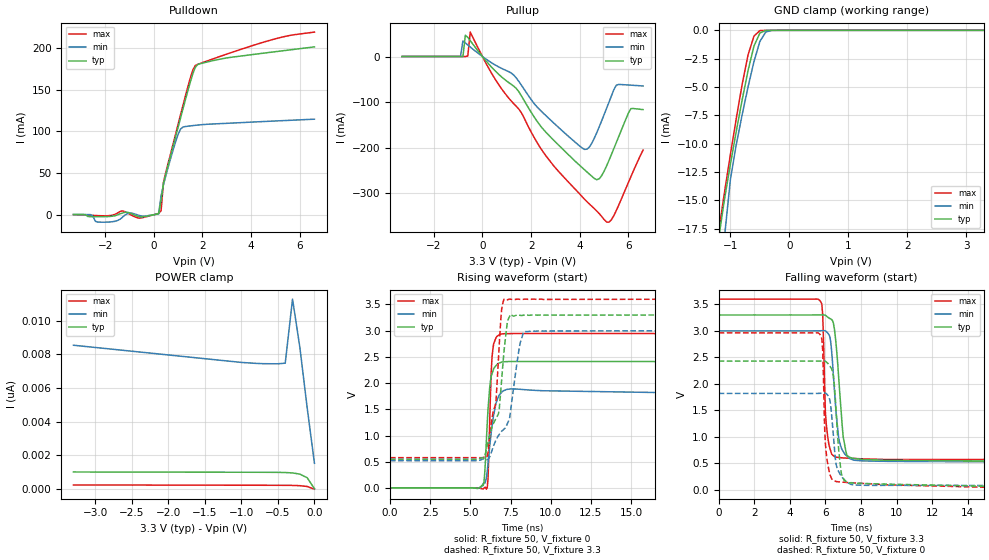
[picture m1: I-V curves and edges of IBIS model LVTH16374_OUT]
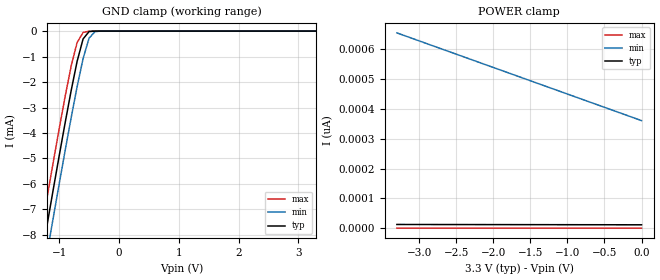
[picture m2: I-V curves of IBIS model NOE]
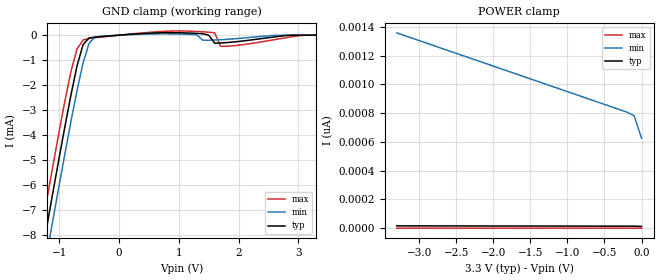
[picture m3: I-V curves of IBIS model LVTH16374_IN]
|   TEXAS INSTRUMENTS INCORPORATED
|   Standard Linear and Logic
|   IBIS Model of SN74LVTH16374
|   3.3V ABT 16-BIT  EDGE-TRIGGERED D-TYPE FLIP-FLOPS
|   WITH 3-STATE OUTPUTS
|   SSOP 48 PIN PACKAGE (DL)
|   TSSOP 48 PIN PACKAGE (DGG)
[IBIS Ver]   2.1
[Comment char]   |_char
[File Name]   sn74lvth16374.ibs
[File Rev]   1.0
[Date]   06-12-2000
[Source]   Data created from HSPICE simulations at TI ,SLL.
[Notes]   The following is an IBIS list for LVTH16374
   - All test data contained in this file are derived from hspice
   (tm) simulations.
   - This file may be incomplete or may not be fully compliant
   with the IBIS specification. It will be replaced with a
   version that is IBIS Revision 3.2 compliant and is complete
   and accurate. Please email all questions and comments to
   sllibis@ti.com.
|   -For Questions or Comments please mailto:sllibis@ti.com
|  [Disclaimer]
|*   Property of Texas Instruments Incorporated.  Unauthorized   *
|*   reproduction and/or distribution is strictly prohibited.   *
|*   This product is protected under copyright law.   *
|*   Created 1995, (C) Copyright 1995, Texas Instruments Inc.,   *
|*   All Rights Reserved   *
|*   UNLESS THERE IS A SIGNED, WRITTEN AGREEMENT TO THE   *
|*   CONTRARY, TEXAS INSTRUMENTS ("TI") IS PROVIDING THE SPICE   *
|*   MODELS "AS IS" AND WITHOUT ANY WARRANTY, EXPRESSED OR   *
|*   IMPLIED.  TI assumes no liability for:   *
|*   1) the accuracy of the IBIS models provided to your   *
|*   company;   *
|*   2) the proper functioning of these IBIS models in your   *
|*   design or for any resulting applications; or   *
|*   3) infringement of patents, copyrights or intellectual   *
|*   property rights resulting from your use of these   *
|*   IBIS models.   *
|*   TI provides IBIS Models as a service to our customers.   *
|*   You and your company shall not distribute, sell or give   *
|*   these models to anyone else without prior written   *
|*   permission from TI.   *
|*   TI reserves the right to make changes to our products or   *
|*   to discontinue any semiconductor product or service   *
|*   without notice, and advises our customers to obtain the   *
|*   latest version of relevant information to verify, before   *
|*   placing orders, that the information being relied on is   *
|*   current.   *
|*   Please be aware that your receipt and use of the IBIS   *
|*   information provided shall serve as acceptance of these   *
|*   terms and conditions.  If you do not accept these terms,   *
|*   you should return or destroy the IBIS models and any   *
|*   other accompanying information immediately.   *
[Component]   LVTH16374_DL
[manufacturer]   Texas   Instruments,   Inc.
[Package]
|   typ   min   max
R_pkg   0.048   0.038   0.053
L_pkg   6.046nH   5.084nH   7.968nH
C_pkg   0.813pF   0.569pF   1.157pF
[Pin]   signal_name   model_name   R_pin   L_pin   C_pin
1   1NOE   NOE   0.046   7.968nH   1.017pF
2   1Q1   LVTH16374_OUT   0.044   7.299nH   1.157pF
3   1Q2   LVTH16374_OUT   0.043   6.765nH   1.058pF
4   GND   GND   0.041   6.269nH   0.933pF
5   1Q3   LVTH16374_OUT   0.038   5.856nH   0.829pF
6   1Q4   LVTH16374_OUT   0.046   5.802nH   0.79pF
7   VCC   POWER   0.05   5.656nH   0.738pF
8   1Q5   LVTH16374_OUT   0.053   5.5nH   0.643pF
9   1Q6   LVTH16374_OUT   0.052   5.304nH   0.606pF
10   GND   GND   0.053   5.189nH   0.583pF
11   1Q7   LVTH16374_OUT   0.051   5.084nH   0.569pF
12   1Q8   LVTH16374_OUT   0.053   5.862nH   0.833pF
13   2Q1   LVTH16374_OUT   0.053   5.862nH   0.833pF
14   2Q2   LVTH16374_OUT   0.051   5.084nH   0.569pF
15   GND   GND   0.053   5.189nH   0.583pF
16   2Q3   LVTH16374_OUT   0.052   5.304nH   0.606pF
17   2Q4   LVTH16374_OUT   0.053   5.5nH   0.643pF
18   VCC   POWER   0.05   5.656nH   0.738pF
19   2Q5   LVTH16374_OUT   0.046   5.802nH   0.79pF
20   2Q6   LVTH16374_OUT   0.038   5.856nH   0.829pF
21   GND   GND   0.041   6.269nH   0.933pF
22   2Q7   LVTH16374_OUT   0.043   6.765nH   1.058pF
23   2Q8   LVTH16374_OUT   0.044   7.299nH   1.157pF
24   2NOE   NOE   0.046   7.968nH   1.017pF
25   2CLK   CLK   0.046   7.968nH   1.017pF
26   2D8   LVTH16374_IN   0.044   7.299nH   1.157pF
27   2D7   LVTH16374_IN   0.043   6.765nH   1.058pF
28   GND   GND   0.041   6.269nH   0.933pF
29   2D6   LVTH16374_IN   0.038   5.856nH   0.829pF
30   2D5   LVTH16374_IN   0.046   5.802nH   0.79pF
31   VCC   POWER   0.05   5.656nH   0.738pF
32   2D4   LVTH16374_IN   0.053   5.5nH   0.643pF
33   2D3   LVTH16374_IN   0.052   5.304nH   0.606pF
34   GND   LVTH16374_IN   0.053   5.189nH   0.583pF
35   2D2   LVTH16374_IN   0.051   5.084nH   0.569pF
36   2D1   LVTH16374_IN   0.053   5.862nH   0.833pF
37   1D8   LVTH16374_IN   0.053   5.862nH   0.833pF
38   1D7   LVTH16374_IN   0.051   5.084nH   0.569pF
39   GND   GND   0.053   5.189nH   0.583pF
40   1D6   LVTH16374_IN   0.052   5.304nH   0.606pF
41   1D5   LVTH16374_IN   0.053   5.5nH   0.643pF
42   VCC   POWER   0.05   5.656nH   0.738pF
43   1D4   LVTH16374_IN   0.046   5.802nH   0.79pF
44   1D3   LVTH16374_IN   0.038   5.856nH   0.829pF
45   GND   GND   0.041   6.269nH   0.933pF
46   1D2   LVTH16374_IN   0.043   6.765nH   1.058pF
47   1D1   LVTH16374_IN   0.044   7.299nH   1.157pF
48   1CLK   CLK   0.046   7.967nH   1.017pF
[Component]   LVTH16374_DGG
[manufacturer]   Texas   Instruments,   Inc.
[Package]
|   typ   min   max
R_pkg   0.056   0.039   0.068
L_pkg   3.39nH   3.078nH   3.995nH
C_pkg   0.52pF   0.414pF   0.668pF
[Pin]   signal_name   model_name   R_pin   L_pin   C_pin
1   1NOE   NOE   0.039   3.987nH   0.654pF
2   1Q1   LVTH16374_OUT   0.047   3.725nH   0.659pF
3   1Q2   LVTH16374_OUT   0.059   3.692nH   0.604pF
4   GND   GND   0.068   3.675nH   0.606pF
5   1Q3   LVTH16374_OUT   0.055   3.473nH   0.547pF
6   1Q4   LVTH16374_OUT   0.056   3.402nH   0.497pF
7   VCC   POWER   0.057   3.3nH   0.492pF
8   1Q5   LVTH16374_OUT   0.056   3.189nH   0.455pF
9   1Q6   LVTH16374_OUT   0.058   3.154nH   0.449pF
10   GND   GND   0.058   3.094nH   0.436pF
11   1Q7   LVTH16374_OUT   0.058   3.078nH   0.424pF
12   1Q8   LVTH16374_OUT   0.06   3.081nH   0.414pF
13   2Q1   LVTH16374_OUT   0.061   3.097nH   0.416pF
14   2Q2   LVTH16374_OUT   0.06   3.126nH   0.427pF
15   GND   GND   0.061   3.158nH   0.44pF
16   2Q3   LVTH16374_OUT   0.058   3.173nH   0.45pF
17   2Q4   LVTH16374_OUT   0.056   3.189nH   0.455pF
18   VCC   POWER   0.056   3.265nH   0.49pF
19   2Q5   LVTH16374_OUT   0.054   3.322nH   0.492pF
20   2Q6   LVTH16374_OUT   0.052   3.388nH   0.544pF
21   GND   GND   0.064   3.591nH   0.605pF
22   2Q7   LVTH16374_OUT   0.059   3.677nH   0.612pF
23   2Q8   LVTH16374_OUT   0.046   3.678nH   0.668pF
24   2NOE   NOE   0.041   3.979nH   0.659pF
25   2CLK   CLK   0.04   3.995nH   0.658pF
26   2D8   LVTH16374_IN   0.046   3.69nH   0.662pF
27   2D7   LVTH16374_IN   0.057   3.649nH   0.602pF
28   GND   GND   0.066   3.615nH   0.602pF
29   2D6   LVTH16374_IN   0.055   3.447nH   0.547pF
30   2D5   LVTH16374_IN   0.054   3.326nH   0.492pF
31   VCC   POWER   0.055   3.239nH   0.488pF
32   2D4   LVTH16374_IN   0.056   3.183nH   0.454pF
33   2D3   LVTH16374_IN   0.057   3.144nH   0.447pF
34   GND   LVTH16374_IN   0.058   3.099nH   0.436pF
35   2D2   LVTH16374_IN   0.059   3.086nH   0.425pF
36   2D1   LVTH16374_IN   0.06   3.081nH   0.414pF
37   1D8   LVTH16374_IN   0.061   3.097nH   0.415pF
38   1D7   LVTH16374_IN   0.06   3.119nH   0.427pF
39   GND   GND   0.06   3.144nH   0.439pF
40   1D6   LVTH16374_IN   0.056   3.13nH   0.446pF
41   1D5   LVTH16374_IN   0.057   3.208nH   0.456pF
42   VCC   POWER   0.056   3.247nH   0.487pF
43   1D4   LVTH16374_IN   0.054   3.328nH   0.491pF
44   1D3   LVTH16374_IN   0.053   3.413nH   0.546pF
45   GND   GND   0.066   3.609nH   0.606pF
46   1D2   LVTH16374_IN   0.058   3.689nH   0.607pF
47   1D1   LVTH16374_IN   0.047   3.727nH   0.662pF
48   1CLK   CLK   0.04   3.978nH   0.655pF
| Models and submodels in the file (4): LVTH16374_OUT (3-state), NOE (Input), CLK (Input), LVTH16374_IN (Input)
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|   Model LVTH16374  OUTPUT
[Model]   LVTH16374_OUT
|Signals
Model_type  3-state
Polarity   Inverting
Enable   Active-Low
Vmeas= 1.5V
Cref = 50pf
Rref = 500
Vref = 0V
| variable   typ   min   max
C_comp   9p   NA   NA
[Temperature Range]   50   100   0
[Voltage range]   3.3   3   3.6
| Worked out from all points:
|   slope of the pulldown table from 0 to 0.495 V, typ, clamps not added: 10.1 ohm
|   slope of the pullup table from 0 to 0.495 V, typ, clamps not added: 16.5 ohm
|   GND clamp passes 1 mA (typ) near -0.57 V on its own axis
|   rising waveform, R_fixture 50, V_fixture 0: 20-80 % time 277ps typ, 419ps min, 179ps max; typ from 0.006 V to 2.41 V
|   falling waveform, R_fixture 50, V_fixture 3.3: 20-80 % time 374ps typ, 358ps min, 188ps max; typ from 3.3 V to 0.55 V
|   rising waveform, R_fixture 50, V_fixture 3.3: 20-80 % time 864ps typ, 1.17ns min, 573ps max; typ from 0.551 V to 3.3 V
|   falling waveform, R_fixture 50, V_fixture 0: 20-80 % time 319ps typ, 365ps min, 212ps max; typ from 2.43 V to 0.007 V
|Process range|   weak   strong
[Pullup]
|   50C:3.3V:   100C:3V:weak   0C:3.6V:strong
|   Voltage   I(typ)   I(min)   I(max)
-3.3V     70.42uA    59uA       80.74uA
-900mV    69.34uA    46.54uA    79.72uA
-800mV    62.99uA    34.29mA    79.64uA
-600mV    42.05mA    25.32mA    1.074mA
-500mV    34.8mA     20.93mA    53.66mA
2.5V      -159.8mA   -124.4mA   -210mA
4.2V      -248.9mA   -204mA     -313.7mA
4.7V      -270.6mA   -167mA     -339.4mA
5.1V      -240.3mA   -113.9mA   -363.5mA
5.5V      -188.9mA   -63.03mA   -338.3mA
6.1V      -114.4mA   -62.91mA   -263.8mA
6.6V      -116.6mA   -64.67mA   -205.4mA
[Pulldown]
|   50C:3.3V:   100C:3V:weak   0C:3.6V:strong
|   Voltage   I(typ)   I(min)   I(max)
-3.3V     150.2uA    119.6uA    -26.2uA
-2.6V     -2.425mA   -37.9uA    -725.3uA
-2.1V     -2.537mA   -9.091mA   -1.41mA
-1V       2.11mA     1.676mA    595.7uA
100mV     466uA      364uA      606.5uA
200mV     1.181mA    1.049mA    1.431mA
300mV     16.78mA    22.44mA    4.721mA
400mV     37.71mA    36.03mA    39.25mA
1.1V      116mA      102.7mA    119.8mA
1.6V      168.5mA    106.7mA    173.1mA
1.8V      179.9mA    107.4mA    180.2mA
6.6V      201.1mA    114.4mA    218.9mA
[GND Clamp]
|   50C:3.3V:   100C:3V:weak   0C:3.6V:strong
|   Voltage   I(typ)   I(min)   I(max)
-3.3V     -662mA     -678mA     -636.5mA
-1.2V     -18.38mA   -28.03mA   -17.77mA
-1.1V     -14.88mA   -18.2mA    -14.27mA
-1V       -11.81mA   -13.15mA   -10.94mA
-900mV    -8.89mA    -10.05mA   -7.747mA
-800mV    -6.107mA   -7.421mA   -4.744mA
-700mV    -3.525mA   -4.972mA   -2.153mA
-600mV    -1.383mA   -2.744mA   -502.1uA
-500mV    -239uA     -981uA     -22.49uA
-400mV    -11.4uA    -147.9uA   -442.5nA
-300mV    -354.7nA   -8.957uA   -12.95nA
3.3V      26.9pA     11.28nA    -1.648nA
[POWER Clamp]
|   50C:3.3V:   100C:3V:weak   0C:3.6V:strong
|   Voltage   I(typ)   I(min)   I(max)
-3.3V     1.02nA     8.541nA    250.4pA
-1V       1.005nA    7.52nA     235.5pA
-700mV    1.003nA    7.447nA    233.1pA
-400mV    989.2pA    7.477nA    228.8pA
-300mV    964.8pA    11.28nA    223.7pA
-200mV    893.6pA    8.419nA    208.7pA
-100mV    680.6pA    4.843nA    160.5pA
0V        26.89pA    1.537nA    1.183pA
[ramp]
| variable   typ   min   max
dV/dt_r   1.4516E+00/2.7334E-10  1.1375E+00/4.5853E-10  1.7801E+00/1.7492E-10
dV/dt_f   1.6506E+00/3.7039E-10  1.4842E+00/3.5176E-10  1.8209E+00/1.8477E-10
[Rising Waveform]
R_fixture = 50
V_fixture = 0
V_fixture_min = 0
V_fixture_max = 0
L_fixture = 0nH
C_fixture = 0pF
|   50C:3.3V:   100C:3V:weak   0C:3.6V:strong
|   Time   V(typ)   V(min)   V(max)
0s        5.704mV    5.196mV    5.998mV
5.5ns     -4.685mV   -3.573mV   93.54uV
5.85ns    122mV      98.04mV    -1.216mV
6ns       923.4mV    194.5mV    -20.69mV
6.1ns     1.504V     468.7mV    184.4mV
6.25ns    2.035V     925mV      1.767V
6.35ns    2.182V     1.189V     2.503V
6.5ns     2.301V     1.469V     2.791V
6.9ns     2.396V     1.809V     2.936V
50ns      2.411V     1.802V     2.946V
[Falling Waveform]
R_fixture = 50
V_fixture = 3.3
V_fixture_min = 3
V_fixture_max = 3.6
L_fixture = 0nH
C_fixture = 0pF
|   50C:3.3V:   100C:3V:weak   0C:3.6V:strong
|   Time   V(typ)   V(min)   V(max)
0s        3.3V       3V         3.6V
5.7ns     3.301V     3.002V     3.57V
5.85ns    3.302V     3.005V     3.294V
6ns       3.294V     3V         1.453V
6.05ns    3.281V     2.987V     1.231V
6.3ns     3.224V     2.786V     726.3mV
6.6ns     2.748V     1.454V     611.1mV
7ns       997mV      719.1mV    597.2mV
7.65ns    586.8mV    553.1mV    586.7mV
50ns      549.7mV    520.7mV    579.1mV
[Rising Waveform]
R_fixture = 50
V_fixture = 3.3
V_fixture_min = 3
V_fixture_max = 3.6
L_fixture = 0nH
C_fixture = 0pF
|   50C:3.3V:   100C:3V:weak   0C:3.6V:strong
|   Time   V(typ)   V(min)   V(max)
0s        550.7mV    521.9mV    579.8mV
6.05ns    811.7mV    540.1mV    607.8mV
6.6ns     1.33V      921.7mV    1.676V
6.75ns    1.416V     1.001V     2.472V
6.95ns    2.074V     1.084V     3.416V
7.1ns     2.622V     1.125V     3.599V
7.5ns     3.313V     1.464V     3.601V
8.05ns    3.296V     2.686V     3.599V
8.35ns    3.298V     2.984V     3.6V
50ns      3.3V       3V         3.6V
[Falling Waveform]
R_fixture = 50
V_fixture = 0
V_fixture_min = 0
V_fixture_max = 0
L_fixture = 0nH
C_fixture = 0pF
|   50C:3.3V:   100C:3V:weak   0C:3.6V:strong
|   Time   V(typ)   V(min)   V(max)
0s        2.428V     1.817V     2.962V
5.7ns     2.43V      1.819V     2.932V
5.85ns    2.431V     1.824V     2.611V
5.95ns    2.428V     1.825V     1.208V
6.05ns    2.412V     1.812V     683.2mV
6.4ns     2.233V     1.218V     186mV
6.6ns     1.492V     476.9mV    150.8mV
6.9ns     296.2mV    251.8mV    140.9mV
7.35ns    126.3mV    112.2mV    131.3mV
50ns      6.986mV    7.066mV    7.474mV
|   LVTH16374 INPUT
[Model]   NOE
| Signals
Model_type  Input
Vinl = 0.8V
Vinh = 2.0V
| variable   typ   min   max
C_comp   3p   NA   NA
[Temperature Range]   50   100   0
[Voltage range]   3.3   3   3.6
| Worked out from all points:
|   GND clamp passes 1 mA (typ) near -0.68 V on its own axis
|Process range|   weak   strong
[GND Clamp]
|   50C:3.3V:   100C:3V:weak   0C:3.6V:strong
|   Voltage   I(typ)   I(min)   I(max)
-3.3V     -36.95mA   -38.01mA   -35.9mA
-1.3V     -8.944mA   -10.05mA   -7.862mA
-1.2V     -7.582mA   -8.693mA   -6.503mA
-1.1V     -6.233mA   -7.342mA   -5.159mA
-900mV    -3.6mA     -4.691mA   -2.565mA
-800mV    -2.345mA   -3.409mA   -1.382mA
-700mV    -1.19mA    -2.185mA   -453.1uA
-600mV    -309.3uA   -1.081mA   -54.51uA
-500mV    -19.64uA   -278uA     -2.59uA
-400mV    -750.2nA   -21.97uA   -121.9nA
3.3V      11.96pA    386.7pA    737.7fA
[POWER Clamp]
|   50C:3.3V:   100C:3V:weak   0C:3.6V:strong
|   Voltage   I(typ)   I(min)   I(max)
-3.3V     13.06pA    653.1pA    765.1fA
-1.5V     12.46pA    493.3pA    752.3fA
-800mV    12.23pA    431.1pA    746.9fA
0V        11.96pA    360.1pA    740.3fA
|   LVTH16374 INPUT
[Model]   LVTH16374_IN
| Signals
Model_type  Input
Vinl = 0.8V
Vinh = 2.0V
| variable   typ   min   max
C_comp   3p   NA   NA
[Temperature Range]   50   100   0
[Voltage range]   3.3   3   3.6
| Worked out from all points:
|   GND clamp passes 1 mA (typ) near -0.67 V on its own axis
|Process range|   weak   strong
[GND Clamp]
|   50C:3.3V:   100C:3V:weak   0C:3.6V:strong
|   Voltage   I(typ)   I(min)   I(max)
-3.3V     -36.95mA   -38.02mA   -35.9mA
-1.3V     -8.951mA   -10.06mA   -7.871mA
-1.2V     -7.59mA    -8.699mA   -6.513mA
-1.1V     -6.242mA   -7.35mA    -5.172mA
-800mV    -2.365mA   -3.423mA   -1.425mA
-700mV    -1.223mA   -2.204mA   -552uA
-600mV    -376.8uA   -1.11mA    -193.1uA
-500mV    -112.6uA   -327.6uA   -130.3uA
-300mV    -58.01uA   -41.81uA   -77.25uA
1.5V      1.985uA    -203.1uA   119.7uA
1.8V      -297.4uA   -168uA     -446.8uA
3.3V      12.85pA    825.8pA    -984.2pA
[POWER Clamp]
|   50C:3.3V:   100C:3V:weak   0C:3.6V:strong
|   Voltage   I(typ)   I(min)   I(max)
-3.3V     16.59pA    1.358nA    770.1fA
-200mV    14.72pA    807.7pA    746.7fA
-100mV    14.61pA    783.2pA    745.8fA
0V        12.85pA    626.2pA    740.7fA
